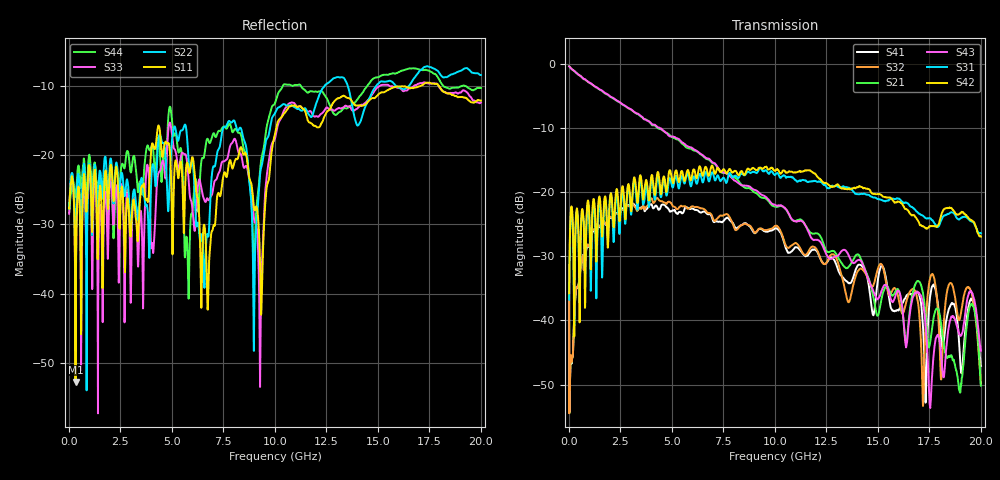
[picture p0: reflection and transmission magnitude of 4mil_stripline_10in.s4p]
! FILE: C:\Archive\Backplane\4-mil striplines\4mil_stripline_10in.s4p
! SMA ->1inch 21mil width microstrip -> 10 inch 4-mil width stripline -> 1 inch 21mil width microstrip -> SMA
! Port 1 -> Port 2, Port 3 -> Port 4
! 10/8/08
# MHz S DB R 50.00
! FREQ  S11  S12  S13  S14
!  S21  S22  S23  S24
!  S31  S32  S33  S34
!  S41  S42  S43  S44
!  DB  ANG  DB  ANG  DB  ANG  DB  ANG
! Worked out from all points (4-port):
!   2000 points, 10 MHz to 20 GHz, reference 50 ohm
!   strongest paths, dB at 10 MHz, 5.01 GHz, 10.01 GHz, 15.01 GHz, 20 GHz:
!     S42: -35.8, -18.1, -16.7, -20.3, -26.9
!     S31: -36.8, -19.1, -17.3, -21.1, -26.4
!     S43: -0.4, -11.3, -22.0, -36.6, -44.7
!     S21: -0.3, -11.4, -22.2, -39.2, -50.2
!     S32: -31.3, -22.0, -25.3, -31.8, -49.8
!     S41: -32.5, -22.9, -25.7, -33.4, -47.1
!   lowest |S11| = -52.7 dB at 320 MHz (marker M1), VSWR 1.00, Z = 50 - j0.231 ohm
!   |S11| at or under -10 dB: start of sweep to 17.11 GHz; 17.95 GHz to end of sweep
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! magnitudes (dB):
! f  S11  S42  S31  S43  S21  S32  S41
! 10 MHz  -27.6  -35.8  -36.8  -0.4  -0.3  -31.3  -32.5
! 320 MHz  -52.7  -25.6  -26.1  -1.3  -1.3  -36.1  -36.1
! 4.31 GHz  -16.1  -16.9  -17.6  -9.9  -10.0  -21.0  -22.5
! 8.06 GHz  -20.8  -16.7  -17.5  -18.2  -17.8  -25.8  -25.5
! 9.34 GHz  -42.8  -16.2  -16.4  -20.4  -20.8  -25.7  -25.8
! 10.69 GHz  -13.0  -16.7  -17.6  -23.4  -23.5  -28.6  -29.4
! 20 GHz  -12.1  -26.9  -26.4  -44.7  -50.2  -49.8  -47.1
